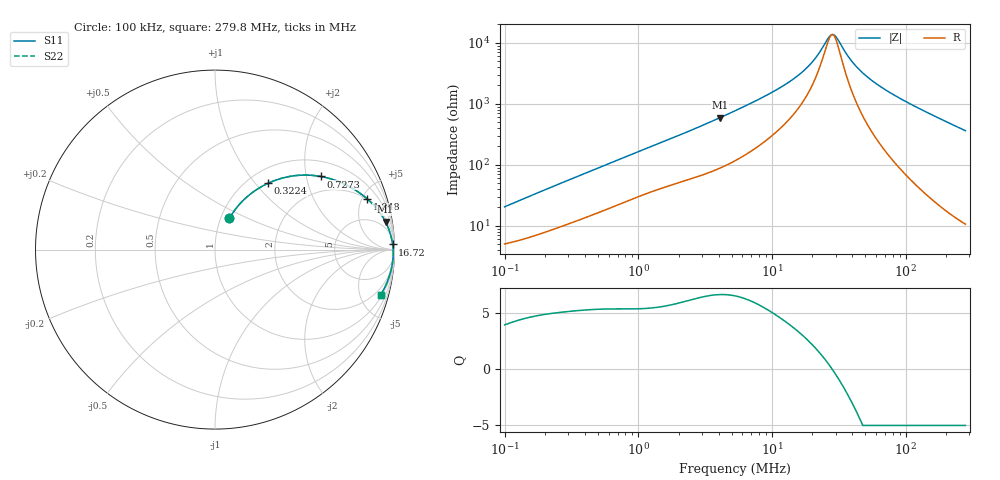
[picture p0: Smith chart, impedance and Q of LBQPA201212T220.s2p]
! LBQPA201212T220  S-PARAMETER MODEL  ( General Type )
! Model Generated by TAIYO YUDEN Corporation (http://www.ty-top.com)
! Version 1.0
! TAIYO YUDEN Control No. 191025NI43SB-FBB
! Copyright(c) 2019 TAIYO YUDEN CO.,LTD. All Rights Reserved.
! Product Description (link to TY-COMPAS)
! https://ds.yuden.co.jp/TYCOMPAS/or/detail?pn=LBQPA201212T220K&u=M
! Products Name : Inductors
! Characteristics :
!  Inductance : 22 uH , SRF(min) : 16 MHz , DC Resistance(max) : 4.81 Ohm
!  Rated Current : Saturation :170 mA , Temp Rise : 145 mA (20 degC)
!  Case Size : 2.0 x 1.25 / 0.079 x 0.049 [mm/inch] , Thickness : 1.25 / 0.049 [mm/inch]
!  (Conditions: Temperature = 25 degC , DC Bias Current/Voltage = 0A / 0V)
! External Node Assignments :
!  1  o---GGG---o  2
! GND o---------o GND
! Frequency Range : 0.1MHz  -  279.750408MHz  [ 402 STEP ]
# MHz S RI R 50
! Freq[MHz].  S11 Real  S11 Imag  S21 Real  S21 Imag  S12 Real  S12 Imag  S22 Real  S22 Imag
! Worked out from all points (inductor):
!   401 points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, 100 kHz to 279.8 MHz, reference 50 ohm
!   read as one part in series: L = 31.2 uH near 104 kHz
!   highest Q = 6.63 at 4.087 MHz (marker M1), where L = 22.8 uH
!   self-resonance near 28 MHz
!   S11 on the Smith chart (normalised r, x): 100 kHz: 1.10, +0.40; 322.4 kHz: 1.23, +1.17; 727.3 kHz: 1.45, +2.43; 1.848 MHz: 1.96, +5.53; 16.72 MHz: 21, +62; 279.8 MHz: 1.21, -7.23
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0.1  0.0807 0.1735  0.9193 -0.1735  0.9193 -0.1735  0.0807 0.1735
0.18498  0.1599 0.2769  0.8401 -0.2769  0.8401 -0.2769  0.1599 0.2769
0.322403  0.2967 0.3701  0.7033 -0.3701  0.7033 -0.3701  0.2967 0.3701
0.377863  0.348 0.3903  0.652 -0.3903  0.652 -0.3903  0.348 0.3903
0.727265  0.5881 0.4076  0.4119 -0.4076  0.4119 -0.4076  0.5881 0.4076
1.427803  0.7937 0.324  0.2063 -0.324  0.2063 -0.324  0.7937 0.324
1.847942  0.8495 0.2813  0.1505 -0.2813  0.1505 -0.2813  0.8495 0.2813
4.08663  0.9501 0.155  0.0499 -0.155  0.0499 -0.155  0.9501 0.155
5.289144  0.9651 0.1222  0.0349 -0.1222  0.0349 -0.1222  0.9651 0.1222
10.80425  0.9848 0.0563  0.0152 -0.0563  0.0152 -0.0563  0.9848 0.0563
16.71734  0.9898 0.0286  0.0102 -0.0286  0.0102 -0.0286  0.9898 0.0286
19.9857  0.9911 0.0186  0.00893 -0.0186  0.00893 -0.0186  0.9911 0.0186
22.51236  0.9918 0.0121  0.00823 -0.0121  0.00823 -0.0121  0.9918 0.0121
26.9137  0.9926 0.00253  0.00744 -0.00253  0.00744 -0.00253  0.9926 0.00253
29.13675  0.9928 -0.00175  0.00718 0.00175  0.00718 0.00175  0.9928 -0.00175
30.92373  0.993 -0.00498  0.00703 0.00498  0.00703 0.00498  0.993 -0.00498
37.7104  0.9932 -0.0161  0.00678 0.0161  0.00678 0.0161  0.9932 -0.0161
44.19738  0.9931 -0.0255  0.00688 0.0255  0.00688 0.0255  0.9931 -0.0255
56.07892  0.9924 -0.0409  0.00761 0.0409  0.00761 0.0409  0.9924 -0.0409
75.51853  0.9902 -0.0636  0.00983 0.0636  0.00983 0.0636  0.9902 -0.0636
136.9498  0.9775 -0.127  0.0225 0.127  0.0225 0.127  0.9775 -0.127
279.7504  0.9226 -0.2529  0.0774 0.2529  0.0774 0.2529  0.9226 -0.2529
